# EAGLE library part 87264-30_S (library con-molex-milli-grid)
RECEPTACAL
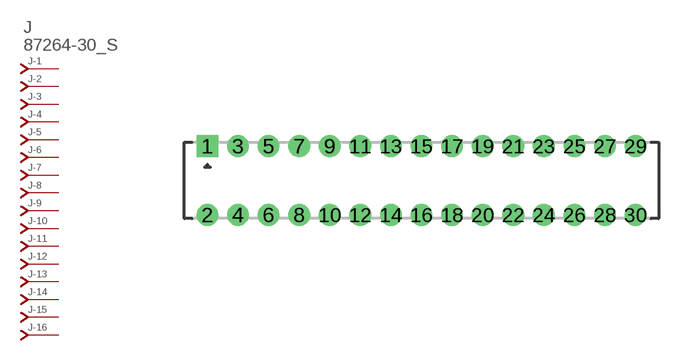
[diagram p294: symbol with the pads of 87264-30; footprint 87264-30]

Designator prefix J; gates -1=J-NV -2=J-N -3=J-N -4=J-N -5=J-N -6=J-N -7=J-N -8=J-N -9=J-N -10=J-N -11=J-N -12=J-N -13=J-N -14=J-N -15=J-N -16=J-N -17=J-N -18=J-N -19=J-N -20=J-N -21=J-N -22=J-N -23=J-N -24=J-N -25=J-N -26=J-N -27=J-N -28=J-N -29=J-N -30=J-N

## 87264-30_S  [87264-30]
1  -1:J  pas
2  -2:J  pas
3  -3:J  pas
4  -4:J  pas
5  -5:J  pas
6  -6:J  pas
7  -7:J  pas
8  -8:J  pas
9  -9:J  pas
10  -10:J  pas
11  -11:J  pas
12  -12:J  pas
13  -13:J  pas
14  -14:J  pas
15  -15:J  pas
16  -16:J  pas
17  -17:J  pas
18  -18:J  pas
19  -19:J  pas
20  -20:J  pas
21  -21:J  pas
22  -22:J  pas
23  -23:J  pas
24  -24:J  pas
25  -25:J  pas
26  -26:J  pas
27  -27:J  pas
28  -28:J  pas
29  -29:J  pas
30  -30:J  pas

## Footprint 87264-30 (pad centres in mm)
RECEPTACAL Dual Row, Side Entry
drill 0.914 square: 1 -14,2.25
drill 0.914: 2 -14,-2.25; 3 -12,2.25; 4 -12,-2.25; 5 -10,2.25; 6 -10,-2.25; 7 -8,2.25; 8 -8,-2.25; 9 -6,2.25; 10 -6,-2.25; 11 -4,2.25; 12 -4,-2.25; 13 -2,2.25; 14 -2,-2.25; 15 0,2.25; 16 0,-2.25; 17 2,2.25; 18 2,-2.25; 19 4,2.25; 20 4,-2.25; 21 6,2.25; 22 6,-2.25; 23 8,2.25; 24 8,-2.25; 25 10,2.25; 26 10,-2.25; 27 12,2.25; 28 12,-2.25; 29 14,2.25; 30 14,-2.25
